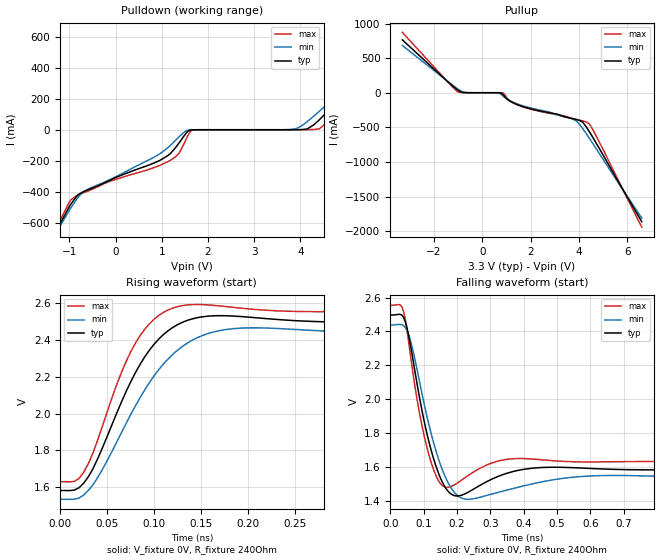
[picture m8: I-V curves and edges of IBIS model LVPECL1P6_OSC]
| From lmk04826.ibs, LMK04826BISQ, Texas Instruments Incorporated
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|   Model LVPECL1P6V
[Model]   LVPECL1P6_OSC
Model_type   Output
Polarity   Non-Inverting
Vmeas = 2.05
Vref = 1.99
Cref = .3pF
Rref = 240
|   typ   min   max
|   (nom PVT)   (fast PVT)   (slow PVT)
C_comp   0.2109p   0.1807p   0.2310p
|C_comp (Low state)   0.2109p   0.1807p   0.2310p
|C_comp (High state)   0.9933p   0.9197p   1.0724p
[Voltage Range]   3.3   3.15   3.45
[Temperature Range]   45   125   -40
[Pullup Reference]   3.3   3.15   3.45
[Pulldown Reference]   0   0   0
[Power Clamp Reference]   3.3   3.15   3.45
[GND Clamp Reference]   0   0   0
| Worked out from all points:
|   slope of the pulldown table from 0 to 0.495 V, typ, clamps not added: 8.73 ohm
|   falling waveform, V_fixture 0V, R_fixture 240Ohm: 20-80 % time 52.7ps typ, 62.3ps min, 45.2ps max; typ from 2.5 V to 1.58 V
|   rising waveform, V_fixture 0V, R_fixture 240Ohm: 20-80 % time 50ps typ, 61ps min, 41.8ps max; typ from 1.58 V to 2.5 V
[Pulldown]
|   Voltage   I(typ)   I(min)   I(max)
-3.3V     -1.869A    -1.737A    -2.051A
-1.29V    -659.3mA   -667.3mA   -647.5mA
-1.003V   -497mA     -520.8mA   -467.3mA
-825mV    -422.7mA   -440mA     -420.4mA
1.175V    -155.7mA   -103.7mA   -198.5mA
1.373V    -85.35mA   -46.2mA    -151.1mA
1.66V     -569.6uA   -270.8uA   -2.008mA
3.887V    106.5uA    6.161mA    2.469uA
4.155V    6.485mA    54.36mA    475.7uA
4.412V    65.2mA     120mA      6.277mA
5.145V    293.7mA    319.5mA    257.9mA
6.59V     761.2mA    723.2mA    811.3mA
[Pullup]
|   Voltage   I(typ)   I(min)   I(max)
-3.3V     764.4mA    683.9mA    873mA
-983.4mV  30.09mA    49.29mA    9.236mA
-686.4mV  508.5uA    3.353mA    377.6uA
561mV     -3.199uA   -263.1uA   -15.17nA
848.1mV   -23.43mA   -44.45mA   -1.6mA
1.115V    -113.4mA   -110mA     -110.4mA
1.531V    -182.7mA   -172.9mA   -185.6mA
3.739V    -374.5mA   -381.3mA   -374.9mA
4.125V    -421.7mA   -506.1mA   -405.1mA
4.392V    -544.4mA   -641.7mA   -441.8mA
4.986V    -896.2mA   -959.4mA   -816.1mA
6.59V     -1.865A    -1.813A    -1.943A
[Ramp]
R_load = 240
|   typ   min   max
dV/dt_r   0.548292/4.99905e-11   0.541543/6.09757e-11   0.55397/4.17605e-11
dV/dt_f   0.548346/5.2725e-11   0.5416/6.22718e-11   0.553999/4.51898e-11
[Falling Waveform]
V_fixture = 0V
V_fixture_min = 0V
V_fixture_max = 0V
R_fixture = 240Ohm
C_fixture = 0F
|   Time   V(typ)   V(min)   V(max)
0s        2.496V     2.437V     2.553V
35ps      2.496V     2.439V     2.543V
55ps      2.375V     2.38V      2.337V
80ps      2.091V     2.176V     1.999V
110ps     1.794V     1.896V     1.713V
165ps     1.477V     1.539V     1.479V
225ps     1.441V     1.408V     1.536V
375ps     1.575V     1.474V     1.648V
630ps     1.587V     1.547V     1.629V
1.9ns     1.582V     1.535V     1.63V
[Rising Waveform]
V_fixture = 0V
V_fixture_min = 0V
V_fixture_max = 0V
R_fixture = 240Ohm
C_fixture = 0F
|   Time   V(typ)   V(min)   V(max)
0s        1.583V     1.535V     1.631V
15ps      1.585V     1.535V     1.632V
25ps      1.622V     1.558V     1.681V
40ps      1.756V     1.654V     1.858V
65ps      2.061V     1.895V     2.221V
85ps      2.267V     2.087V     2.423V
105ps     2.405V     2.239V     2.533V
135ps     2.505V     2.381V     2.589V
205ps     2.521V     2.465V     2.565V
1.9ns     2.497V     2.438V     2.554V
